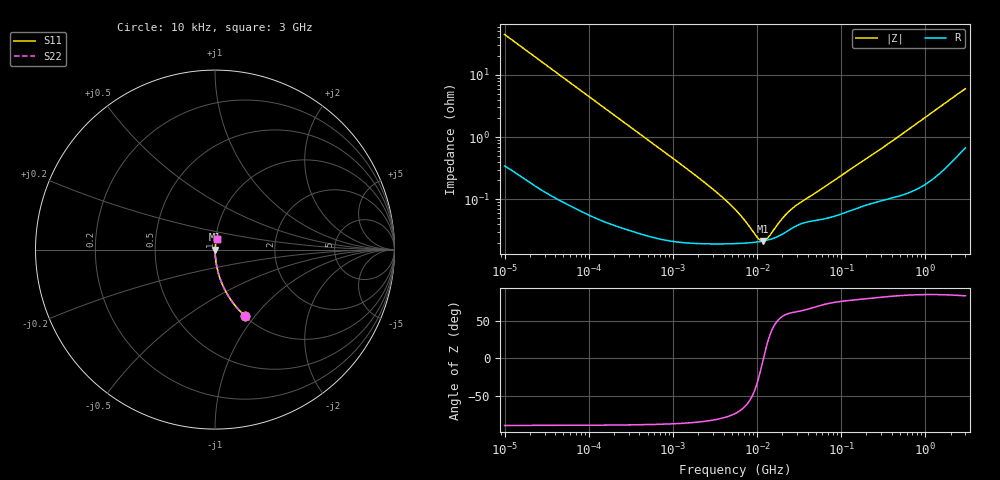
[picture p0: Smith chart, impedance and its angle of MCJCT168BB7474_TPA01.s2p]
! MCJCT168BB7474_TPA01  S-PARAMETER MODEL  ( Standard Model )
! Model Generated by TAIYO YUDEN Corporation (http://www.ty-top.com)
! Version 1.0
! TAIYO YUDEN Control No. 220601
! Copyright(c) 2015 TAIYO YUDEN CO.,LTD. All Rights Reserved.
! Product Description (link to TY-COMPAS)
! https://ds.yuden.co.jp/TYCOMPAS/or/detail?pn=MCJCT168BB7474KTPA01&u=M
! Products Name : Multilayer Ceramic Capacitors
! Characteristics :
!  Capacitance : 0.47 [uF] , Rated Voltage : 25 [V] , TCC : X7R
!  Case Size : 1.6 x 0.8 / 0.063 x 0.031 [mm/inch] , Thickness : 0.8 / 0.031 [mm/inch]
!  (Conditions: Temperature = 25 [degC] , DC Bias Voltage = 0 [V])
! External Node Assignments :
!  1  o---| |---o  2
! GND o---------o GND
! Frequency Range : 10kHz  -  3GHz  [ 401 STEP ]
# MHZ S RI R 50
! Freq[MHz].  S11 Real  S11 Imag  S21 Real  S21 Imag  S12 Real  S12 Imag  S22 Real  S22 Imag
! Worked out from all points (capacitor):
!   401 points, 10 kHz to 3 GHz, reference 50 ohm
!   read as one part in series: C = 356 nF near 10.65 kHz
!   lowest |Z| = 21.2 mohm at 11.67 MHz (marker M1)
!   series resonance near 11.95 MHz, so ESL is about 500 pH
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0.01  0.1684 -0.3704  0.8316 0.3704  0.8316 0.3704  0.1684 -0.3704
0.014599  0.0879 -0.2791  0.9121 0.2791  0.9121 0.2791  0.0879 -0.2791
0.021995  0.0415 -0.1952  0.9585 0.1952  0.9585 0.1952  0.0415 -0.1952
0.040039  0.0135 -0.1108  0.9865 0.1108  0.9865 0.1108  0.0135 -0.1108
0.082683  0.0036 -0.0544  0.9964 0.0544  0.9964 0.0544  0.0036 -0.0544
0.199902  0.000893 -0.0227  0.9991 0.0227  0.9991 0.0227  0.000893 -0.0227
0.683653  0.000274 -0.00667  0.9997 0.00667  0.9997 0.00667  0.000274 -0.00667
2.652321  0.000194 -0.00164  0.9998 0.00164  0.9998 0.00164  0.000194 -0.00164
3.996065  0.000192 -0.00102  0.9998 0.00102  0.9998 0.00102  0.000192 -0.00102
5.477226  0.000193 -0.000661  0.9998 0.000661  0.9998 0.000661  0.000193 -0.000661
7.048603  0.000196 -0.000424  0.9998 0.000424  0.9998 0.000424  0.000196 -0.000424
9.97066  0.000205 -0.00014  0.9998 0.00014  0.9998 0.00014  0.000205 -0.00014
10.95979  0.000208 -6.62e-05  0.9998 6.62e-05  0.9998 6.62e-05  0.000208 -6.62e-05
11.67315  0.000211 -1.76e-05  0.9998 1.76e-05  0.9998 1.76e-05  0.000211 -1.76e-05
12.43293  0.000215 3.09e-05  0.9998 -3.09e-05  0.9998 -3.09e-05  0.000215 3.09e-05
13.66633  0.000222 0.000104  0.9998 -0.000104  0.9998 -0.000104  0.000222 0.000104
19.33182  0.000267 0.000379  0.9997 -0.000379  0.9997 -0.000379  0.000267 0.000379
24.87798  0.000328 0.00058  0.9997 -0.00058  0.9997 -0.00058  0.000328 0.00058
31.02164  0.000387 0.000747  0.9996 -0.000747  0.9996 -0.000747  0.000387 0.000747
45.28751  0.000446 0.00108  0.9996 -0.00108  0.9996 -0.00108  0.000446 0.00108
374.4521  0.00108 0.00794  0.9989 -0.00794  0.9989 -0.00794  0.00108 0.00794
3000  0.0101 0.0586  0.9899 -0.0586  0.9899 -0.0586  0.0101 0.0586
